| TEXAS INSTRUMENTS INCORPORATED
| Standard Linear and Logic Group
| IBIS Model of SN74CBTLV3383
| LOW-VOLTAGE 10-BIT FET BUS-EXCHANGE SWITCH
| This file contains package information for the following:
|  SOIC 24-pin (DW) package as [Component] CBTLV3383_DW
|  TSSOP 24-pin (PW) package as [Component] CBTLV3383_PW
|  TVSOP 24-pin (DGV) package as [Component] CBTLV3383_DGV
|  SSOP 24-pin (DBQ) package as [Component] CBTLV3383_DBQ
| This device can be powered at the following Vccs:
|  3.3 volt Vcc
|  2.5 volt Vcc
| This file provides unique models under the [Model Selector] for each Vcc.
| For operation at a specific Vcc, select the appropriate model after each
| [Model Selector] keyword.
[IBIS Ver]   3.2
[Comment char]  |_char
[File Name]   sn74cbtlv3383.ibs
[File Rev]   1.1 | x_die
[Date]   April 4, 2005
[Source]   Data created from TI-SPICE simulations at TI-SLL.
[Notes]   The following is an IBIS list for the CBTLV3383.
   Please contact sllibis@ti.com with questions and
   comments concerning SLL IBIS models.
   - FILE REV HISTORY
   - 1.1 Release IBIS file on 04/04/05
   - Power clamp data deleted as there is no power-clamp diode.
   - Non-monotonic data due to FET characteristics.
[Disclaimer] Property of Texas Instruments Incorporated.  Unauthorized
   reproduction and/or distribution is strictly prohibited.
   This product is protected under copyright law.
   Created  2005, (C) Copyright  2005, Texas Instruments
   Incorporated, All Rights Reserved
   UNLESS THERE IS A SIGNED, WRITTEN AGREEMENT TO THE
   CONTRARY, TEXAS INSTRUMENTS (TI) IS PROVIDING THE IBIS
   MODELS  AND WITHOUT ANY WARRANTY, EXPRESSED OR
   IMPLIED.  TI assumes no liability for:
   1) the accuracy of the IBIS models provided to your
   company;
   2) the proper functioning of these IBIS Models in your
   design or for any resulting applications; or
   3) infringement of patents, copyrights or intellectual
   property rights resulting from your use of these IBIS
   models.
   TI provides IBIS Models as a service to our customers.
   You and your company shall not distribute, sell or give
   these models to anyone else without prior written
   permission from TI.
   TI reserves the right to make changes to our products or
   to discontinue any semiconductor product or service
   without notice, and advises our customers to obtain the
   latest version of relevant information to verify, before
   placing orders, that the information being relied on is
   current.
   Please be aware that your receipt and use of the IBIS
   information provided shall serve as acceptance of these
   terms and conditions.  If you do not accept these terms,
   you should return or destroy the IBIS models and any
   other accompanying information immediately.
| Component CBTLV3383_DW 24-pin SOIC
[Component]   CBTLV3383_DW
[Manufacturer]   Texas Instruments, Inc.
[Package]
|   typ   min   max
R_pkg   3.700e-02   3.000e-02   4.700e-02
L_pkg   5.146e-09   3.993e-09   6.885e-09
C_pkg   7.580e-13   5.120e-13   1.067e-12
[Pin]   signal_name   model_name   R_pin   L_pin   C_pin
1   NBE   CBTLV3383_IN   3.900e-02   6.885e-09   1.067e-12
2   1B1   CBTLV3383_IO   4.200e-02   5.950e-09   9.580e-13
3   1A1   CBTLV3383_IO   4.700e-02   5.317e-09   7.910e-13
4   1A2   CBTLV3383_IO   3.100e-02   4.651e-09   6.110e-13
5   1B2   CBTLV3383_IO   3.000e-02   3.993e-09   5.120e-13
6   2B1   CBTLV3383_IO   3.000e-02   4.083e-09   6.110e-13
7   2A1   CBTLV3383_IO   3.000e-02   4.083e-09   6.110e-13
8   2A2   CBTLV3383_IO   3.000e-02   3.993e-09   5.120e-13
9   2B2   CBTLV3383_IO   3.100e-02   4.652e-09   6.110e-13
10   3B1   CBTLV3383_IO   4.700e-02   5.317e-09   7.910e-13
11   3A1   CBTLV3383_IO   4.200e-02   5.950e-09   9.590e-13
12   GND   GND   3.900e-02   6.885e-09   1.067e-12
13   BX   CBTLV3383_IN   3.900e-02   6.885e-09   1.067e-12
14   3A2   CBTLV3383_IO   4.200e-02   5.950e-09   9.590e-13
15   3B2   CBTLV3383_IO   4.700e-02   5.317e-09   7.910e-13
16   4B1   CBTLV3383_IO   3.100e-02   4.652e-09   6.110e-13
17   4A1   CBTLV3383_IO   3.000e-02   3.993e-09   5.120e-13
18   4A2   CBTLV3383_IO   3.000e-02   4.083e-09   6.100e-13
19   4B2   CBTLV3383_IO   3.000e-02   4.083e-09   6.100e-13
20   5B1   CBTLV3383_IO   3.000e-02   3.993e-09   5.120e-13
21   5A1   CBTLV3383_IO   3.100e-02   4.651e-09   6.110e-13
22   5A2   CBTLV3383_IO   4.700e-02   5.317e-09   7.910e-13
23   5B2   CBTLV3383_IO   4.200e-02   5.950e-09   9.580e-13
24   VCC   POWER   3.900e-02   6.885e-09   1.067e-12
| Component CBTLV3383_PW 24-pin TSSOP
[Component]   CBTLV3383_PW
[Manufacturer]   Texas Instruments, Inc.
[Package]
|   typ   min   max
R_pkg   3.900e-02   3.000e-02   4.600e-02
L_pkg   2.685e-09   2.367e-09   3.177e-09
C_pkg   3.200e-13   2.520e-13   4.340e-13
[Pin]   signal_name   model_name   R_pin   L_pin   C_pin
1   NBE   CBTLV3383_IN   3.700e-02   3.153e-09   4.340e-13
2   1B1   CBTLV3383_IO   3.400e-02   2.629e-09   3.410e-13
3   1A1   CBTLV3383_IO   3.200e-02   2.860e-09   3.470e-13
4   1A2   CBTLV3383_IO   4.200e-02   2.741e-09   2.900e-13
5   1B2   CBTLV3383_IO   4.600e-02   2.600e-09   2.620e-13
6   2B1   CBTLV3383_IO   4.300e-02   2.414e-09   2.660e-13
7   2A1   CBTLV3383_IO   4.200e-02   2.367e-09   2.620e-13
8   2A2   CBTLV3383_IO   4.400e-02   2.461e-09   2.520e-13
9   2B2   CBTLV3383_IO   4.200e-02   2.543e-09   2.740e-13
10   3B1   CBTLV3383_IO   3.000e-02   2.616e-09   3.320e-13
11   3A1   CBTLV3383_IO   3.700e-02   2.670e-09   3.460e-13
12   GND   GND   3.900e-02   3.177e-09   4.330e-13
13   BX   CBTLV3383_IN   3.700e-02   3.111e-09   4.310e-13
14   3A2   CBTLV3383_IO   3.700e-02   2.656e-09   3.450e-13
15   3B2   CBTLV3383_IO   3.100e-02   2.739e-09   3.400e-13
16   4B1   CBTLV3383_IO   4.200e-02   2.649e-09   2.820e-13
17   4A1   CBTLV3383_IO   4.600e-02   2.532e-09   2.570e-13
18   4A2   CBTLV3383_IO   4.400e-02   2.425e-09   2.660e-13
19   4B2   CBTLV3383_IO   4.400e-02   2.425e-09   2.660e-13
20   5B1   CBTLV3383_IO   4.600e-02   2.532e-09   2.570e-13
21   5A1   CBTLV3383_IO   4.200e-02   2.648e-09   2.820e-13
22   5A2   CBTLV3383_IO   3.100e-02   2.738e-09   3.390e-13
23   5B2   CBTLV3383_IO   3.600e-02   2.653e-09   3.440e-13
24   VCC   POWER   3.700e-02   3.110e-09   4.310e-13
| Component CBTLV3383_DGV 24-pin TVSOP
[Component]   CBTLV3383_DGV
[Manufacturer]   Texas Instruments, Inc.
[Package]
|   typ   min   max
R_pkg   4.300e-02   3.900e-02   4.700e-02
L_pkg   2.601e-09   2.312e-09   3.626e-09
C_pkg   3.580e-13   2.770e-13   5.950e-13
[Pin]   signal_name   model_name   R_pin   L_pin   C_pin
1   NBE   CBTLV3383_IN   4.300e-02   3.625e-09   5.950e-13
2   1B1   CBTLV3383_IO   4.000e-02   2.656e-09   4.020e-13
3   1A1   CBTLV3383_IO   3.900e-02   2.338e-09   3.080e-13
4   1A2   CBTLV3383_IO   4.600e-02   2.354e-09   2.770e-13
5   1B2   CBTLV3383_IO   4.500e-02   2.312e-09   2.850e-13
6   2B1   CBTLV3383_IO   4.700e-02   2.318e-09   2.820e-13
7   2A1   CBTLV3383_IO   4.700e-02   2.318e-09   2.820e-13
8   2A2   CBTLV3383_IO   4.500e-02   2.312e-09   2.850e-13
9   2B2   CBTLV3383_IO   4.600e-02   2.353e-09   2.780e-13
10   3B1   CBTLV3383_IO   3.900e-02   2.338e-09   3.080e-13
11   3A1   CBTLV3383_IO   4.100e-02   2.660e-09   4.020e-13
12   GND   GND   4.300e-02   3.625e-09   5.950e-13
13   BX   CBTLV3383_IN   4.400e-02   3.626e-09   5.940e-13
14   3A2   CBTLV3383_IO   4.000e-02   2.658e-09   4.020e-13
15   3B2   CBTLV3383_IO   3.900e-02   2.343e-09   3.110e-13
16   4B1   CBTLV3383_IO   4.600e-02   2.353e-09   2.780e-13
17   4A1   CBTLV3383_IO   4.500e-02   2.312e-09   2.850e-13
18   4A2   CBTLV3383_IO   4.700e-02   2.319e-09   2.820e-13
19   4B2   CBTLV3383_IO   4.700e-02   2.319e-09   2.820e-13
20   5B1   CBTLV3383_IO   4.500e-02   2.312e-09   2.850e-13
21   5A1   CBTLV3383_IO   4.600e-02   2.353e-09   2.780e-13
22   5A2   CBTLV3383_IO   3.900e-02   2.337e-09   3.080e-13
23   5B2   CBTLV3383_IO   4.000e-02   2.658e-09   4.020e-13
24   VCC   POWER   4.400e-02   3.626e-09   5.950e-13
| Component CBTLV3383_DBQ 24-pin SSOP
[Component]   CBTLV3383_DBQ
[Manufacturer]   Texas Instruments, Inc.
[Package]
|   typ   min   max
R_pkg   4.400e-02   3.100e-02   6.600e-02
L_pkg   3.074e-09   2.348e-09   4.044e-09
C_pkg   3.220e-13   2.340e-13   4.460e-13
[Pin]   signal_name   model_name   R_pin   L_pin   C_pin
1   NBE   CBTLV3383_IN   6.500e-02   4.044e-09   4.290e-13
2   1B1   CBTLV3383_IO   6.600e-02   3.824e-09   4.460e-13
3   1A1   CBTLV3383_IO   3.100e-02   3.011e-09   3.210e-13
4   1A2   CBTLV3383_IO   3.200e-02   2.699e-09   2.590e-13
5   1B2   CBTLV3383_IO   3.500e-02   2.519e-09   2.450e-13
6   2B1   CBTLV3383_IO   3.500e-02   2.348e-09   2.340e-13
7   2A1   CBTLV3383_IO   3.500e-02   2.348e-09   2.340e-13
8   2A2   CBTLV3383_IO   3.500e-02   2.518e-09   2.450e-13
9   2B2   CBTLV3383_IO   3.200e-02   2.699e-09   2.590e-13
10   3B1   CBTLV3383_IO   3.100e-02   3.011e-09   3.210e-13
11   3A1   CBTLV3383_IO   6.600e-02   3.824e-09   4.460e-13
12   GND   GND   6.500e-02   4.044e-09   4.290e-13
13   BX   CBTLV3383_IN   6.500e-02   4.044e-09   4.290e-13
14   3A2   CBTLV3383_IO   6.600e-02   3.824e-09   4.460e-13
15   3B2   CBTLV3383_IO   3.100e-02   3.011e-09   3.210e-13
16   4B1   CBTLV3383_IO   3.200e-02   2.699e-09   2.590e-13
17   4A1   CBTLV3383_IO   3.500e-02   2.518e-09   2.450e-13
18   4A2   CBTLV3383_IO   3.500e-02   2.348e-09   2.340e-13
19   4B2   CBTLV3383_IO   3.500e-02   2.348e-09   2.340e-13
20   5B1   CBTLV3383_IO   3.500e-02   2.518e-09   2.450e-13
21   5A1   CBTLV3383_IO   3.200e-02   2.699e-09   2.590e-13
22   5A2   CBTLV3383_IO   3.100e-02   3.011e-09   3.210e-13
23   5B2   CBTLV3383_IO   6.600e-02   3.824e-09   4.460e-13
24   VCC   POWER   6.500e-02   4.044e-09   4.290e-13
[Series Switch Groups]
| Function Group States
On  1 /   | 1A1-5A1->1B1-5B1 NBE LOW BX LOW
   | 1A2-5A2->1B2-5B2 NBE LOW BX LOW
On  2 /   | 1A1-5A1->1B2-5B2 NBE LOW BX HIGH
   | 1A2-5A2->1B1-5B1 NBE LOW BX HIGH
Off 1 2 /   | NBE HIGH
[Series Pin Mapping]   pin_2   model_name   function_table_group
3   2   CBTLV3383_IO_33_S   1
| 3   2   CBTLV3383_IO_25_S   1
7   6   CBTLV3383_IO_33_S   1
| 7   6   CBTLV3383_IO_25_S   1
11   10   CBTLV3383_IO_33_S   1
| 11   10   CBTLV3383_IO_25_S   1
17   16   CBTLV3383_IO_33_S   1
| 17   16   CBTLV3383_IO_25_S   1
21   20   CBTLV3383_IO_33_S   1
| 21   20   CBTLV3383_IO_25_S   1
4   5   CBTLV3383_IO_33_S   1
| 4   5   CBTLV3383_IO_25_S   1
8   9   CBTLV3383_IO_33_S   1
| 8   9   CBTLV3383_IO_25_S   1
14   15   CBTLV3383_IO_33_S   1
| 14   15   CBTLV3383_IO_25_S   1
18   19   CBTLV3383_IO_33_S   1
| 18   19   CBTLV3383_IO_25_S   1
22   23   CBTLV3383_IO_33_S   1
| 22   23   CBTLV3383_IO_25_S   1
3   5   CBTLV3383_IO_33_S   2
| 3   5   CBTLV3383_IO_25_S   2
7   9   CBTLV3383_IO_33_S   2
| 7   9   CBTLV3383_IO_25_S   2
11   15   CBTLV3383_IO_33_S   2
| 11   15   CBTLV3383_IO_25_S   2
17   19   CBTLV3383_IO_33_S   2
| 17   19   CBTLV3383_IO_25_S   2
21   23   CBTLV3383_IO_33_S   2
| 21   23   CBTLV3383_IO_25_S   2
4   2   CBTLV3383_IO_33_S   2
| 4   2   CBTLV3383_IO_25_S   2
8   6   CBTLV3383_IO_33_S   2
| 8   6   CBTLV3383_IO_25_S   2
14   10   CBTLV3383_IO_33_S   2
| 14   10   CBTLV3383_IO_25_S   2
18   16   CBTLV3383_IO_33_S   2
| 18   16   CBTLV3383_IO_25_S   2
22   20   CBTLV3383_IO_33_S   2
| 22   20   CBTLV3383_IO_25_S   2
| Model CBTLV3383_IN
[Model Selector]   CBTLV3383_IN
CBTLV3383_IN_33   3.3 volt Vcc
CBTLV3383_IN_25   2.5 volt Vcc
| Model CBTLV3383_IO
[Model Selector]   CBTLV3383_IO
CBTLV3383_IO_33   3.3 volt Vcc
CBTLV3383_IO_25   2.5 volt Vcc
| Model CBTLV3383_IO_S
[Model Selector]   CBTLV3383_IO_S
CBTLV3383_IO_33_S   3.3 volt Vcc_S
CBTLV3383_IO_25_S   2.5 volt Vcc_S
[Model]   CBTLV3383_IO_33_S
Model_type  Series_switch
| variable   typ   min   max
C_comp   0   0   0
[Temperature Range]   40   100   -40
| Ambient temperature   25   85   -40
[Voltage range]   3.3   3   3.6
[On]
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[Off]
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[Model]   CBTLV3383_IO_25_S
Model_type  Series_switch
| variable   typ   min   max
C_comp   0   0   0
[Temperature Range]   40   100   -40
| Ambient temperature   25   85   -40
[Voltage range]   2.5   2.3   2.7
[On]
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[Off]
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| Models and submodels in the file (6): CBTLV3383_IN_33 (Input), CBTLV3383_IN_25 (Input), CBTLV3383_IO_33_S (Series_switch), CBTLV3383_IO_33 (Terminator), CBTLV3383_IO_25_S (Series_switch), CBTLV3383_IO_25 (Terminator)
